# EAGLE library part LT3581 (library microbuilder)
LTC3581 - 3.3A Boost/Inverting DC/DC Converter (Boost/SEPIC/Inverting or Flyback) Digikey: LT3581EDE#PBF-ND
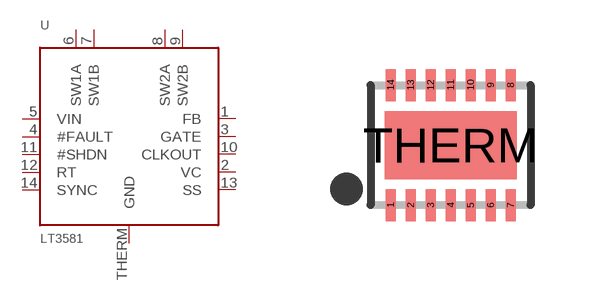
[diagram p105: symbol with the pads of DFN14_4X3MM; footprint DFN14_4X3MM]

Designator prefix U

## LT3581  [DFN14_4X3MM]
1  FB
2  VC
3  GATE
4  #FAULT
5  VIN  pwr
6  SW1A  pwr
7  SW1B  pwr
8  SW2A  pwr
9  SW2B  pwr
10  CLKOUT  out
11  #SHDN
12  RT
13  SS
14  SYNC
THERM  GND  pwr

## Footprint DFN14_4X3MM (pad centres in mm)
14-lead DFN (4.0x3.0mm) Source: http://cds.linear.com/docs/Datasheet/3581f.pdf
smd 0.25 x 0.8: 1 -1.5,-1.5; 2 -1,-1.5; 3 -0.5,-1.5; 4 0,-1.5; 5 0.5,-1.5; 6 1,-1.5; 7 1.5,-1.5; 8 1.5,1.5; 9 1,1.5; 10 0.5,1.5; 11 0,1.5; 12 -0.5,1.5; 13 -1,1.5; 14 -1.5,1.5
smd 3.3 x 1.7: THERM 0,0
